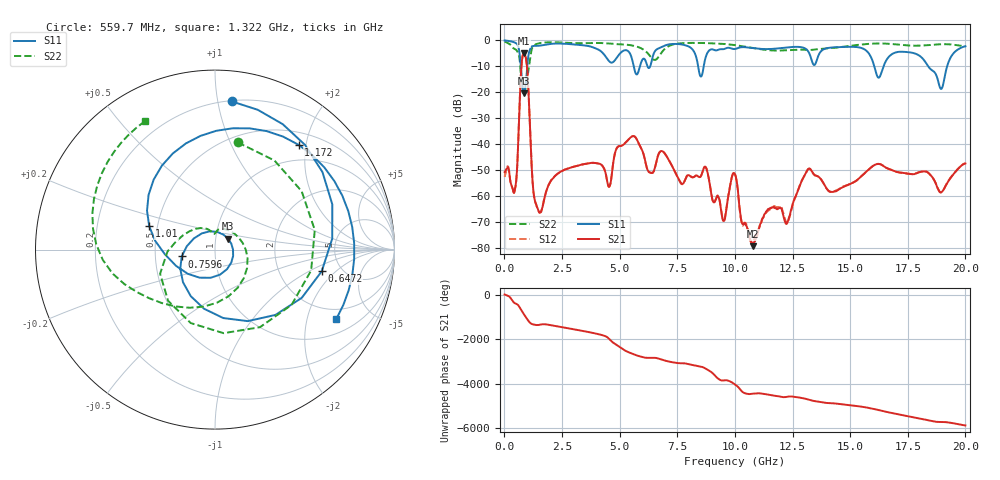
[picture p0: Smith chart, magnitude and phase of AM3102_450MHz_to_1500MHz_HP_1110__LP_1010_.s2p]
!Agilent Technologies,E8364B,MY43040894,A.07.50.67
!Agilent E8364B: A.07.50.67
!Date: Thursday, January 11, 2018 06:44:53
!Correction: S11(Full 2 Port(1,2))
!S21(Full 2 Port(1,2))
!S12(Full 2 Port(1,2))
!S22(Full 2 Port(1,2))
!S2P File: Measurements: S11, S21, S12, S22:
# Hz S  dB  R 50
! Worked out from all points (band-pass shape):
!   1601 points, 10 MHz to 20 GHz, reference 50 ohm
!   highest |S21| = -5.01 dB at 847.1 MHz (marker M1); lowest = -79.2 dB at 10.79 GHz (marker M2)
!   |S21| within 3 dB of the highest: 759.9 MHz to 953.8 MHz (193.9 MHz wide, 22.6 % of centre)
!   lowest |S11| = -20.4 dB at 847.1 MHz (marker M3), VSWR 1.21, Z = 57.4 + j7.11 ohm
!   |S11| at or under -10 dB: 715 MHz to 992.8 MHz (277.8 MHz wide, 32.5 % of centre); 16.05 GHz to 16.45 GHz (404.2 MHz wide, 2.49 % of centre); 18.38 GHz to 19.21 GHz (825.5 MHz wide, 4.39 % of centre)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
!   |S22| runs from -21.2 to -0.5 dB; largest |S21 - S12| = 0.00073
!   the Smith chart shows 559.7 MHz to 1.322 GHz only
!   S11 on the Smith chart (normalised r, x): 559.7 MHz: 0.21, +1.10; 647.2 MHz: 3.53, -1.35; 759.6 MHz: 0.69, -0.05; 1.01 GHz: 0.45, +0.14; 1.172 GHz: 0.71, +1.86; 1.322 GHz: 1.54, -3.03
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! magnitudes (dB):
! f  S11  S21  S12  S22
! 10 MHz  -0.1  -50.7  -52.6  -0.5
! 409.8 MHz  -0.8  -58.7  -59.0  -3.2
! 559.7 MHz  -1.6  -47.9  -48.0  -4.3
! 647.2 MHz  -4.3  -27.5  -27.5  -6.6
! 759.6 MHz  -14.5  -8.0  -8.0  -16.8
! 847.1 MHz  -20.4  -5.0  -5.0  -21.0
! 1.01 GHz  -8.2  -13.7  -13.7  -13.7
! 1.172 GHz  -2.5  -46.2  -46.2  -4.0
! 1.322 GHz  -2.2  -61.6  -61.5  -1.8
! 3.346 GHz  -1.9  -47.8  -47.8  -1.2
! 4.545 GHz  -8.1  -56.4  -56.3  -1.2
! 5.745 GHz  -13.2  -38.1  -38.1  -2.5
! 6.307 GHz  -10.4  -50.8  -50.8  -5.9
! 6.682 GHz  -3.2  -44.0  -43.9  -6.5
! 8.731 GHz  -6.6  -48.8  -48.8  -1.1
! 9.505 GHz  -3.4  -69.5  -68.9  -1.4
! 10.01 GHz  -3.4  -51.5  -51.5  -1.9
! 10.79 GHz  -3.0  -79.2  -77.3  -3.0
! 13.34 GHz  -8.0  -50.4  -50.5  -3.7
! 16.68 GHz  -6.4  -49.5  -49.5  -1.4
! 18.95 GHz  -18.7  -58.4  -58.5  -1.5
! 20 GHz  -2.3  -47.4  -47.3  -2.3
